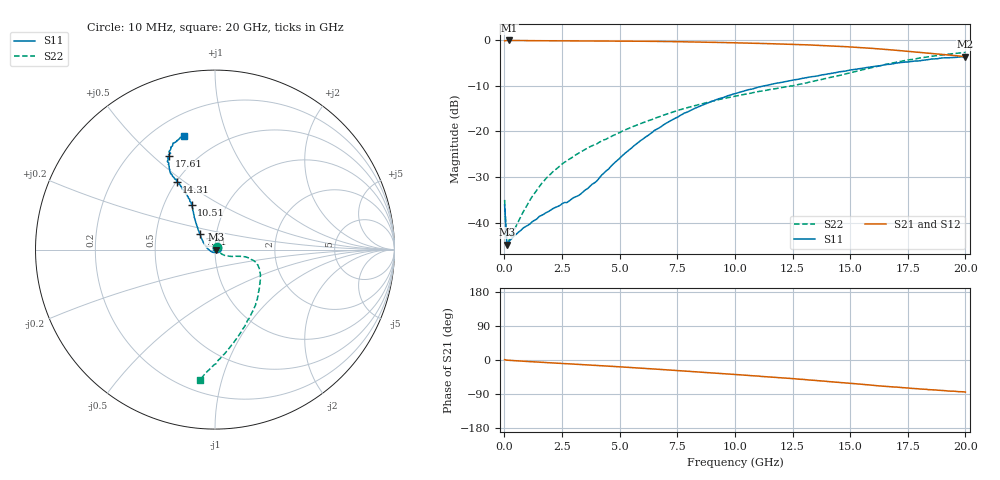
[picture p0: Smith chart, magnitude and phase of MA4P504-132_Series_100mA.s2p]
! AWR Design Environment (9226) Thu Aug 19 02:45:16 2021
! Document = '100mA'
! nPorts: 2, nXvals: 201
# GHz S DB R 50
!Freq DBS11 AngS11 DBS21 AngS21 DBS12 AngS12 DBS22 AngS22
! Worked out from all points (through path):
!   201 points, 10 MHz to 20 GHz, reference 50 ohm
!   highest |S21| = -0.10 dB at 210 MHz (marker M1); lowest = -3.6 dB at 20 GHz (marker M2)
!   group delay of S21, straight-line fit = 11.9 ps
!   lowest |S11| = -44.8 dB at 110 MHz (marker M3), VSWR 1.01, Z = 50.6 + j0.0259 ohm
!   |S11| at or under -10 dB: start of sweep to 11.31 GHz
!   |S22| runs from -45.1 to -2.7 dB; largest |S21 - S12| = 0.032
!   S11 on the Smith chart (normalised r, x): 10 MHz: 1.03, +0.02; 7.01 GHz: 0.83, +0.15; 10.51 GHz: 0.69, +0.37; 14.31 GHz: 0.50, +0.47; 17.61 GHz: 0.36, +0.56; 20 GHz: 0.32, +0.71
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0.01  -36.09 30.4  -0.17 1.1  -0.12 0.4  -35.02 55.9
0.11  -44.78 2.5  -0.10 -0.4  -0.09 -0.5  -45.14 2.4
0.21  -44.07 0.4  -0.10 -0.9  -0.09 -0.9  -43.74 1.8
0.81  -41.19 -24.0  -0.13 -3.2  -0.12 -3.1  -37.69 -16.8
1.11  -40.27 -37.2  -0.14 -4.3  -0.13 -4.2  -35.05 -23.5
1.61  -38.41 -58.9  -0.16 -6.0  -0.15 -5.9  -31.46 -28.9
2.51  -35.83 -100.8  -0.19 -9.2  -0.18 -8.9  -27.14 -33.6
2.71  -35.59 -110.1  -0.19 -9.8  -0.18 -9.5  -26.49 -32.6
3.41  -33.29 -143.3  -0.20 -12.3  -0.20 -11.9  -24.23 -30.7
4.01  -30.87 -167.6  -0.21 -14.5  -0.21 -14.0  -22.76 -27.8
5.21  -24.90 158.7  -0.25 -18.9  -0.24 -18.2  -19.78 -22.0
6.71  -19.27 137.1  -0.31 -24.6  -0.30 -23.8  -16.83 -15.1
7.01  -18.24 134.5  -0.33 -25.8  -0.32 -25.0  -16.28 -14.5
8.31  -14.85 125.8  -0.44 -31.0  -0.44 -30.0  -14.31 -13.8
10.01  -11.74 118.3  -0.61 -38.2  -0.60 -36.7  -12.31 -17.7
10.51  -10.97 117.5  -0.67 -40.3  -0.65 -38.7  -11.82 -20.5
13.41  -7.99 118.5  -1.12 -53.4  -1.04 -51.9  -9.02 -47.6
14.31  -7.23 119.4  -1.34 -57.9  -1.22 -56.4  -7.99 -57.7
16.71  -5.32 118.5  -2.13 -70.5  -2.01 -69.0  -5.17 -81.4
17.61  -4.73 116.3  -2.51 -74.6  -2.42 -73.7  -4.30 -87.5
19.01  -3.91 111.6  -3.13 -80.4  -3.15 -80.2  -3.27 -94.1
20  -3.64 105.4  -3.64 -84.6  -3.74 -84.0  -2.72 -96.5
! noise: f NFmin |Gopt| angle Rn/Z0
0.01  0  1  0  2e-20
2.21  0  1  0  2e-20
4.41  0  1  0  2e-20
6.61  0  1  0  2e-20
8.81  0  1  0  2e-20
11.11  0  1  0  2e-20
13.31  0  1  0  2e-20
15.51  0  1  0  2e-20
17.71  0  1  0  2e-20
20  0  1  0  2e-20
